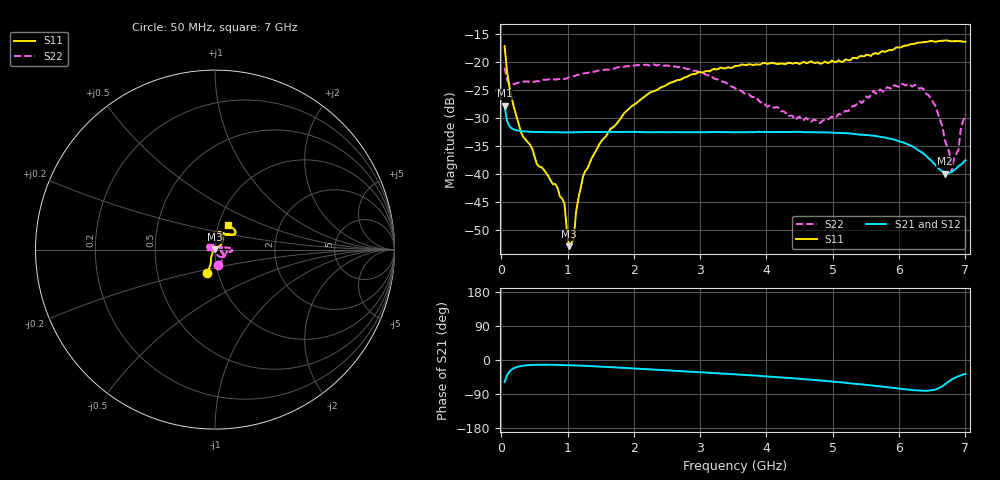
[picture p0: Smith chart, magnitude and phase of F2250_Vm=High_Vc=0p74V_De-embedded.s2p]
! Integrated Device Technology
! Corporate Headquarters
! 6024 Silver Creek Valley Road
! San Jose, CA 95138  USA
! Phone:  1-408-284-8200
! Toll Free:  1-800-223-1366
! Webpage:  http://www.idt.com/
! Timing and RF Division
! 515 Groton Road, Suite 102
! Westford, MA 01886-6024
! Device:  F2250
! Description: Voltage Variable RF Attenuator
! Frequency:  50.0 -  6000.00 MHz
! Package:  3x3 mm Thin QFN Plastic Package: 16 pin
! Ports:  2 RF, 3 DC
!  Pin  1  = GND
!  Pin  2  = NC
!  Pin  3  = RF1  = Port 1
!  Pin  4  = NC
!  Pin  5  = GND
!  Pin  6  = GND
!  Pin  7  = GND
!  Pin  8  = GND
!  Pin  9  = NC
!  Pin 10  = RF2  = Port 2
!  Pin 11  = NC
!  Pin 12  = GND
!  Pin 13  = GND
!  Pin 14  = VCNTRL
!  Pin 15  = VDD
!  Pin 16  = VMODE
! Vcntrl:  0.740 Volts
! Vmode:  +3.300 Volts
! Vdd:  +3.30  Volts
! Current:  1.294 mA
! Data:  The device was measured on a the F2250 evaluation board which has
!  individual transmission lines to the RF pins.  Data was collected
!  using a calibrated network analyzer.  The evaluation board was
!  de-embedded using a TRL calibration technique.
!  The reference plane is the edge of the package pin.
! Misc:  SN 10
!  Action Tracker AT0258
! Date Measured:  2014-11-26
! Date:  2015-10-15  MJV
! Note:
!  Integrated Device Technology supplies this data as a sample of measured
!  data at the package pin for this product.  Your particular data for this
!  product may vary.
!  Data was taken at 25 degrees C.
!  Integrated Device Technology reserves the right to change this data at anytime.
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# GHz S dB R 50
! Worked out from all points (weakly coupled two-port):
!   201 points, 50 MHz to 7 GHz, reference 50 ohm
!   highest |S21| = -27.79 dB at 50 MHz (marker M1); lowest = -40.0 dB at 6.687 GHz (marker M2)
!   lowest |S11| = -53.0 dB at 1.023 GHz (marker M3), VSWR 1.00, Z = 49.8 + j0.162 ohm
!   |S11| at or under -10 dB: start of sweep to end of sweep
!   |S22| runs from -39.7 to -20.4 dB; largest |S21 - S12| = 9.3e-05
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0.05  -17.15 -108.0  -27.79 -58.0  -27.79 -58.0  -20.97 -80.3
0.1195  -24.20 -111.2  -31.43 -31.3  -31.42 -31.3  -23.82 -32.0
0.29325  -32.37 -125.7  -32.34 -16.0  -32.34 -16.0  -23.50 -14.1
0.9535  -45.35 172.6  -32.57 -13.4  -32.59 -13.4  -23.04 -9.2
1.023  -52.96 133.8  -32.59 -13.7  -32.57 -13.7  -22.70 -9.0
1.0925  -51.79 73.7  -32.55 -14.1  -32.55 -14.1  -22.54 -8.9
1.12725  -46.88 52.4  -32.55 -14.3  -32.55 -14.3  -22.37 -9.3
1.2315  -40.55 36.6  -32.53 -15.1  -32.54 -15.1  -22.06 -10.2
1.6485  -31.94 39.6  -32.52 -18.8  -32.51 -18.8  -21.31 -7.7
2.37825  -24.75 46.0  -32.54 -26.0  -32.54 -26.0  -20.49 -2.4
3.525  -20.70 71.3  -32.57 -37.8  -32.55 -37.9  -24.67 10.4
4.4285  -20.15 74.4  -32.48 -48.7  -32.50 -48.7  -30.35 18.7
4.7065  -20.11 71.8  -32.54 -52.5  -32.56 -52.5  -30.31 8.4
5.01925  -19.95 63.1  -32.66 -57.4  -32.64 -57.5  -30.07 -3.2
5.85325  -17.82 40.3  -33.70 -72.3  -33.69 -72.4  -24.64 -33.1
6.3745  -16.42 40.8  -36.41 -81.3  -36.43 -81.3  -24.91 -47.9
6.54825  -16.37 44.5  -38.41 -77.7  -38.43 -77.8  -27.85 -62.1
6.68725  -16.13 47.6  -39.98 -64.8  -39.99 -64.8  -33.86 -77.7
6.75675  -16.21 50.3  -39.82 -56.1  -39.82 -56.1  -36.12 -100.0
6.7915  -16.27 51.1  -39.69 -51.4  -39.70 -51.3  -39.69 -125.2
6.89575  -16.24 56.2  -38.63 -42.9  -38.61 -42.8  -35.69 171.1
7  -16.37 62.2  -37.55 -37.0  -37.53 -37.1  -29.39 154.2
